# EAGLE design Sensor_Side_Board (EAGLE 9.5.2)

## Sheet 1 of 2: Sensor side expansion board for hoop house controller - Inputs
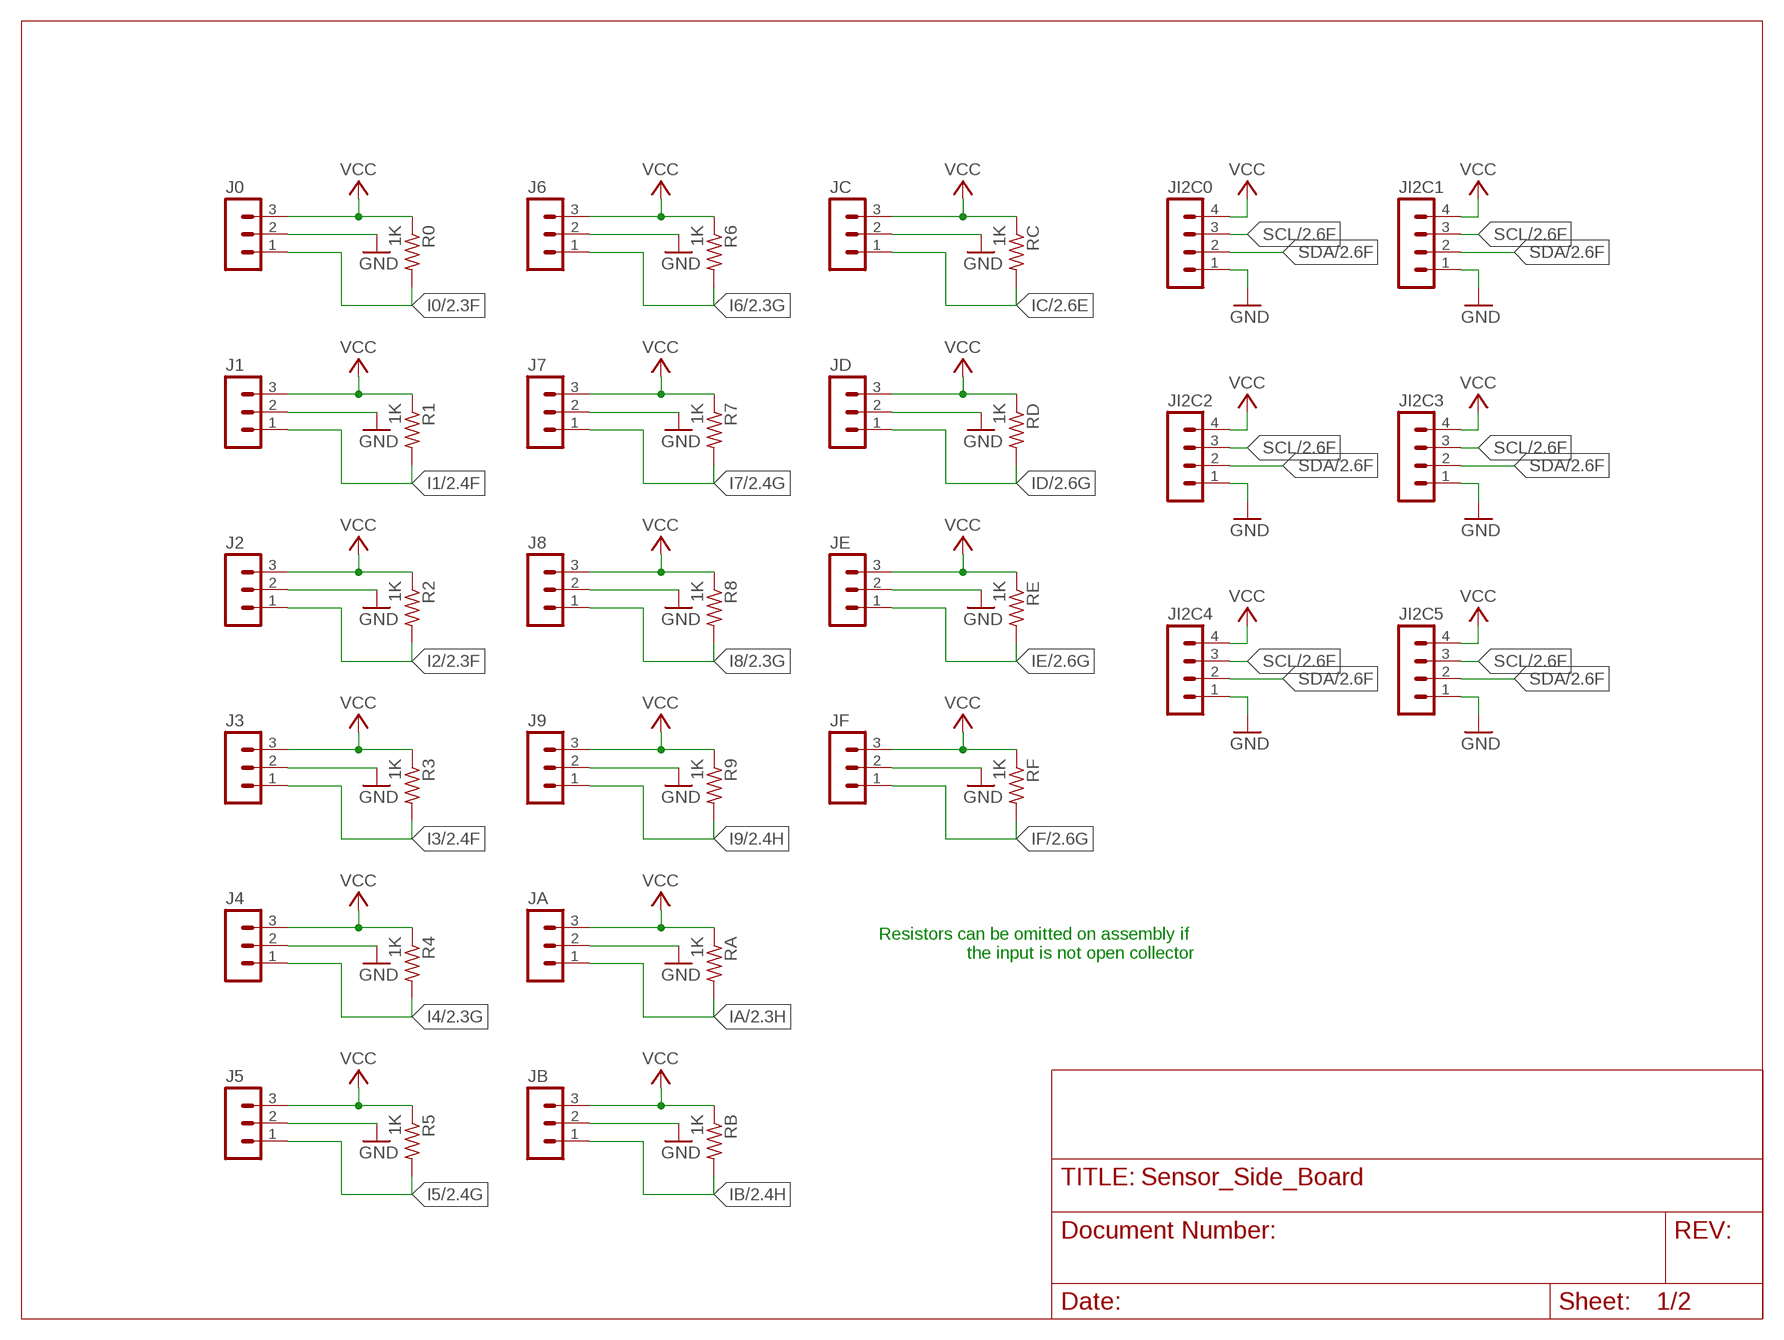
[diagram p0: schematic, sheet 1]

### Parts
J0  MA03-1  [MA03-1]
J1  MA03-1  [MA03-1]
J2  MA03-1  [MA03-1]
J3  MA03-1  [MA03-1]
J4  MA03-1  [MA03-1]
J5  MA03-1  [MA03-1]
J6  MA03-1  [MA03-1]
J7  MA03-1  [MA03-1]
J8  MA03-1  [MA03-1]
J9  MA03-1  [MA03-1]
JA  MA03-1  [MA03-1]
JB  MA03-1  [MA03-1]
JC  MA03-1  [MA03-1]
JD  MA03-1  [MA03-1]
JE  MA03-1  [MA03-1]
JF  MA03-1  [MA03-1]
JI2C0  MA04-1  [MA04-1]
JI2C1  MA04-1  [MA04-1]
JI2C2  MA04-1  [MA04-1]
JI2C3  MA04-1  [MA04-1]
JI2C4  MA04-1  [MA04-1]
JI2C5  MA04-1  [MA04-1]
R0  1K  R-US_0411/15  [0411/15]
R1  1K  R-US_0411/15  [0411/15]
R2  1K  R-US_0411/15  [0411/15]
R3  1K  R-US_0411/15  [0411/15]
R4  1K  R-US_0411/15  [0411/15]
R5  1K  R-US_0411/15  [0411/15]
R6  1K  R-US_0411/15  [0411/15]
R7  1K  R-US_0411/15  [0411/15]
R8  1K  R-US_0411/15  [0411/15]
R9  1K  R-US_0411/15  [0411/15]
RA  1K  R-US_0411/15  [0411/15]
RB  1K  R-US_0411/15  [0411/15]
RC  1K  R-US_0411/15  [0411/15]
RD  1K  R-US_0411/15  [0411/15]
RE  1K  R-US_0411/15  [0411/15]
RF  1K  R-US_0411/15  [0411/15]

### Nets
GND: J0.2 J1.2 J2.2 J3.2 J4.2 J5.2 J6.2 J7.2 J8.2 J9.2 JA.2 JB.2 JC.2 JD.2 JE.2 JF.2 JI2C0.1 JI2C1.1 JI2C2.1 JI2C3.1 JI2C4.1 JI2C5.1 ; also sheet 2
I0: J0.1 R0.2 ; also sheet 2
I1: J1.1 R1.2 ; also sheet 2
I2: J2.1 R2.2 ; also sheet 2
I3: J3.1 R3.2 ; also sheet 2
I4: J4.1 R4.2 ; also sheet 2
I5: J5.1 R5.2 ; also sheet 2
I6: J6.1 R6.2 ; also sheet 2
I7: J7.1 R7.2 ; also sheet 2
I8: J8.1 R8.2 ; also sheet 2
I9: J9.1 R9.2 ; also sheet 2
IA: JA.1 RA.2 ; also sheet 2
IB: JB.1 RB.2 ; also sheet 2
IC: JC.1 RC.2 ; also sheet 2
ID: JD.1 RD.2 ; also sheet 2
IE: JE.1 RE.2 ; also sheet 2
IF: JF.1 RF.2 ; also sheet 2
SCL: JI2C0.3 JI2C1.3 JI2C2.3 JI2C3.3 JI2C4.3 JI2C5.3 ; also sheet 2
SDA: JI2C0.2 JI2C1.2 JI2C2.2 JI2C3.2 JI2C4.2 JI2C5.2 ; also sheet 2
VCC: J0.3 J1.3 J2.3 J3.3 J4.3 J5.3 J6.3 J7.3 J8.3 J9.3 JA.3 JB.3 JC.3 JD.3 JE.3 JF.3 JI2C0.4 JI2C1.4 JI2C2.4 JI2C3.4 JI2C4.4 JI2C5.4 R0.1 R1.1 R2.1 R3.1 R4.1 R5.1 R6.1 R7.1 R8.1 R9.1 RA.1 RB.1 RC.1 RD.1 RE.1 RF.1 ; also sheet 2

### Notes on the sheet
- Resistors can be omitted on assembly if 
  the input is not open collector

## Sheet 2 of 2: Sensor side expansion board for hoop house controller - ESP, optical isolation, and output
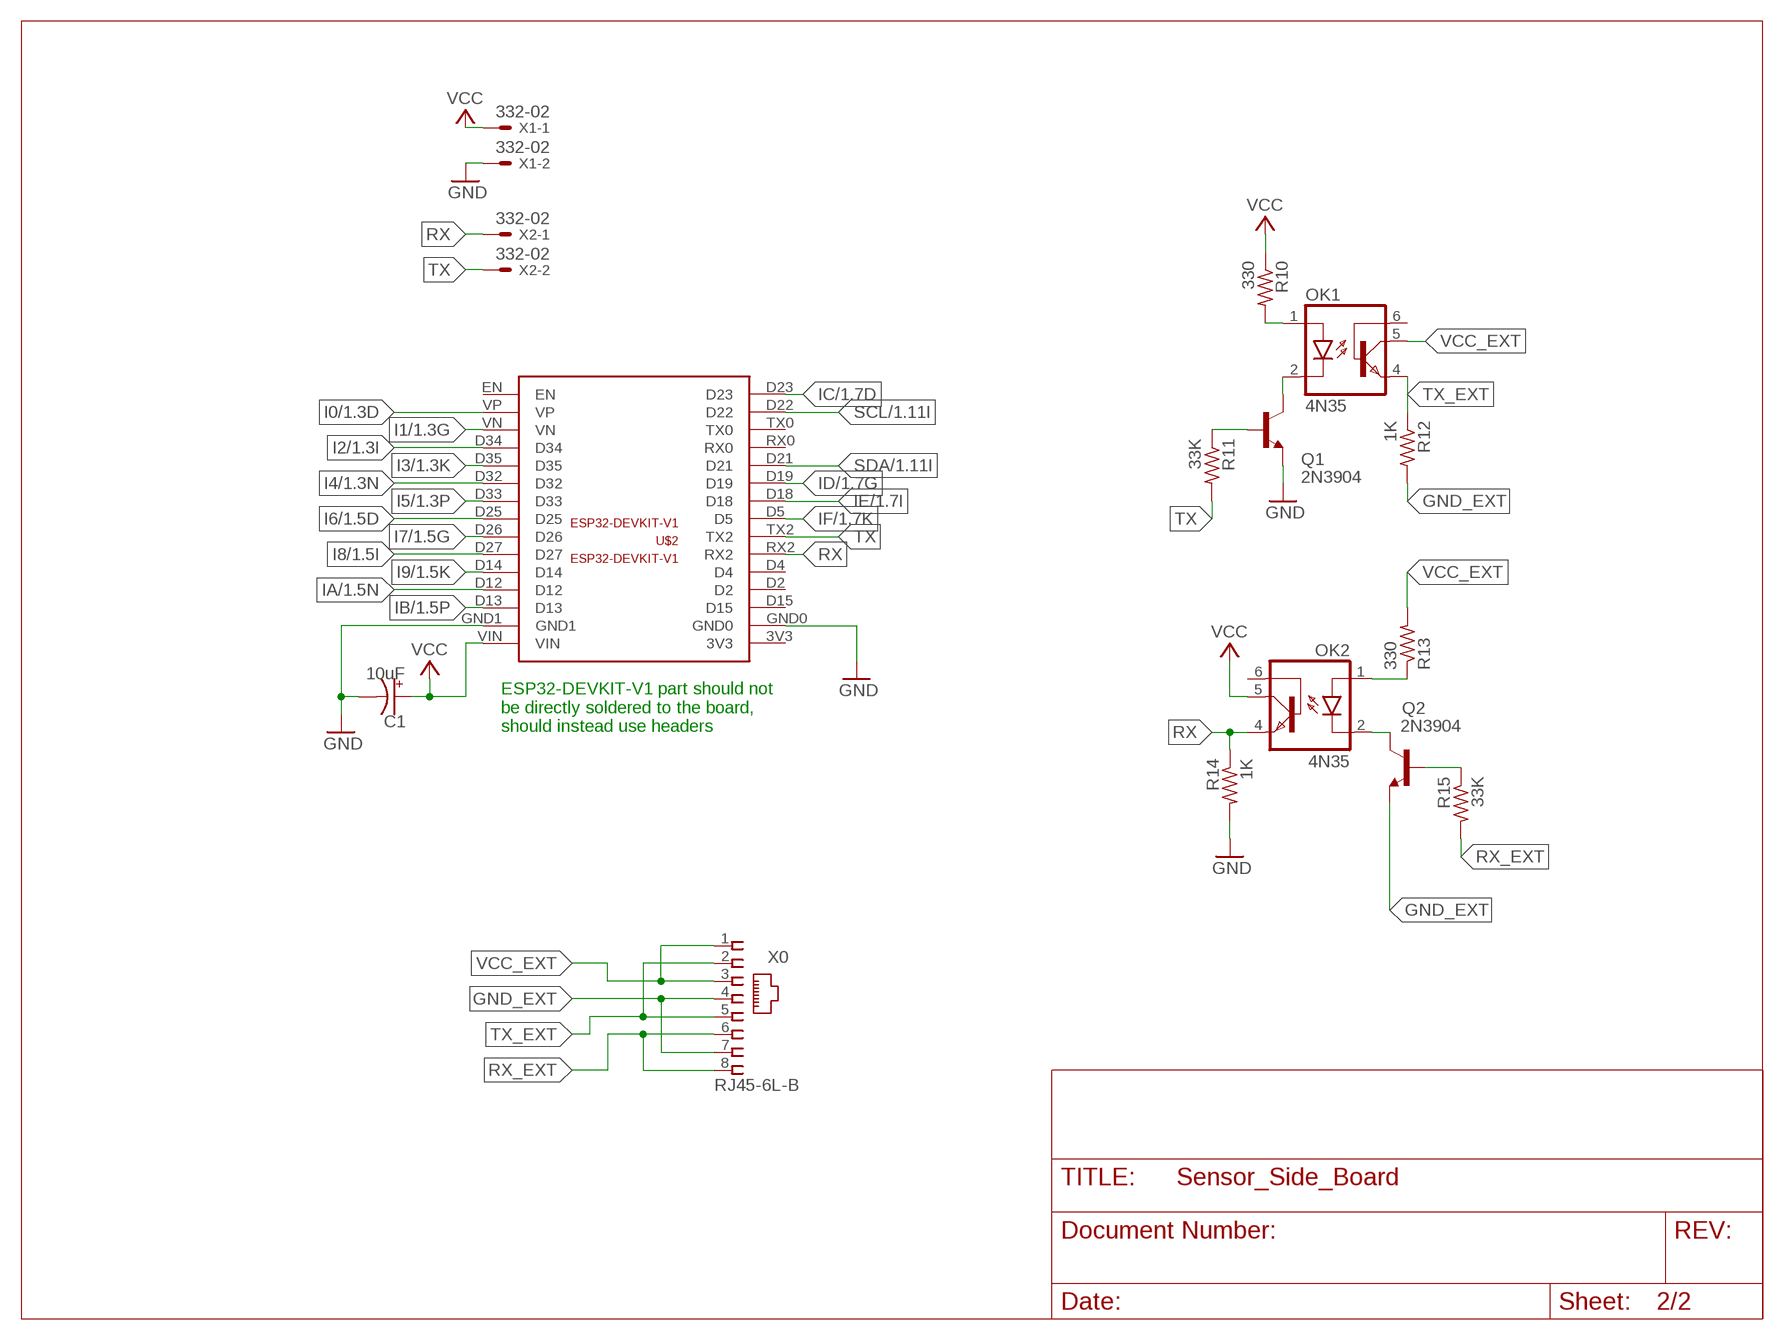
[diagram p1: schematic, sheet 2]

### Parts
C1  10uF  CPOL-USE3.5-10  [E3,5-10]
OK1  4N35  [DIL06]
OK2  4N35  [DIL06]
Q1  2N3904  [TO92]
Q2  2N3904  [TO92]
R10  330  R-US_0411/15  [0411/15]
R11  33K  R-US_0411/15  [0411/15]
R12  1K  R-US_0411/15  [0411/15]
R13  330  R-US_0411/15  [0411/15]
R14  1K  R-US_0411/15  [0411/15]
R15  33K  R-US_0411/15  [0411/15]
U$2  ESP32-DEVKIT-V1  [ESP32-DEVKIT-V1]
X0  RJ45-6L-B  [RJ45-NO-SHIELD]
X1  332-02  [332-02]
X2  332-02  [332-02]

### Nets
GND: C1.- Q1.3(E) R14.2 U$2.GND0 U$2.GND1 X1.2 ; also sheet 1
GND_EXT: Q2.3(E) R12.2 X0.4 X0.7
I0: U$2.VP ; also sheet 1
I1: U$2.VN ; also sheet 1
I2: U$2.D34 ; also sheet 1
I3: U$2.D35 ; also sheet 1
I4: U$2.D32 ; also sheet 1
I5: U$2.D33 ; also sheet 1
I6: U$2.D25 ; also sheet 1
I7: U$2.D26 ; also sheet 1
I8: U$2.D27 ; also sheet 1
I9: U$2.D14 ; also sheet 1
IA: U$2.D12 ; also sheet 1
IB: U$2.D13 ; also sheet 1
IC: U$2.D23 ; also sheet 1
ID: U$2.D19 ; also sheet 1
IE: U$2.D18 ; also sheet 1
IF: U$2.D5 ; also sheet 1
N$6: OK1.1(A) R10.2
N$7: Q1.2(B) R11.1
N$8: OK2.1(A) R13.1
N$9: OK1.2(C) Q1.1(C)
N$13: OK2.2(C) Q2.1(C)
N$14: Q2.2(B) R15.1
RX: OK2.4(EMI) R14.1 U$2.RX2 X2.1
RX_EXT: R15.2 X0.6 X0.8
SCL: U$2.D22 ; also sheet 1
SDA: U$2.D21 ; also sheet 1
TX: R11.2 U$2.TX2 X2.2
TX_EXT: OK1.4(EMI) R12.1 X0.2 X0.5
VCC: C1.+ OK2.5(COL) R10.1 U$2.VIN X1.1 ; also sheet 1
VCC_EXT: OK1.5(COL) R13.2 X0.1 X0.3
Unconnected: OK1.6(BAS) OK2.6(BAS) U$2.3V3 U$2.D2 U$2.D4 U$2.D15 U$2.EN U$2.RX0 U$2.TX0

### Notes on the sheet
- ESP32-DEVKIT-V1 part should not
  be directly soldered to the board,
  should instead use headers

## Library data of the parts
C1 = rcl:CPOL-US: POLARIZED CAPACITOR, American symbol; SPICEPREFIX: C
J0 J1-J9 JA JB JC JD JE JF = con-lstb:MA03-1: PIN HEADER; OC_FARNELL: unknown; OC_NEWARK: unknown
JI2C0 JI2C1-JI2C5 = con-lstb:MA04-1: PIN HEADER; OC_FARNELL: unknown; OC_NEWARK: unknown
OK1 OK2 = optocoupler:4N35: MOTOROLA OPTO COUPLER; MF: FAIRCHILD SEMICONDUCTOR; MPN: 4N35; OC_FARNELL: 1328375; OC_NEWARK: 72K9946
Q1 Q2 = transistor-npn:2N3904: NPN Transistor
R0 R1-R15 RA RB RC RD RE RF = resistor:R-US_: RESISTOR, American symbol
U$2 = FF Hoop House Controller:ESP32-DEVKIT-V1
X0 = con-tycoelectronics:RJ45: CORCOM Modular RJ Jacks No Shield Source: www.tycoelectronics.com .. ENG_DS_1654001_1099_RJ_L_0507.pdf; MPN: RJ45-6L-B; OC_FARNELL: unknown; OC_NEWARK: 16R6090
X1 X2 = con-garry:332-02: 2 Pin - 2mm Dual Row

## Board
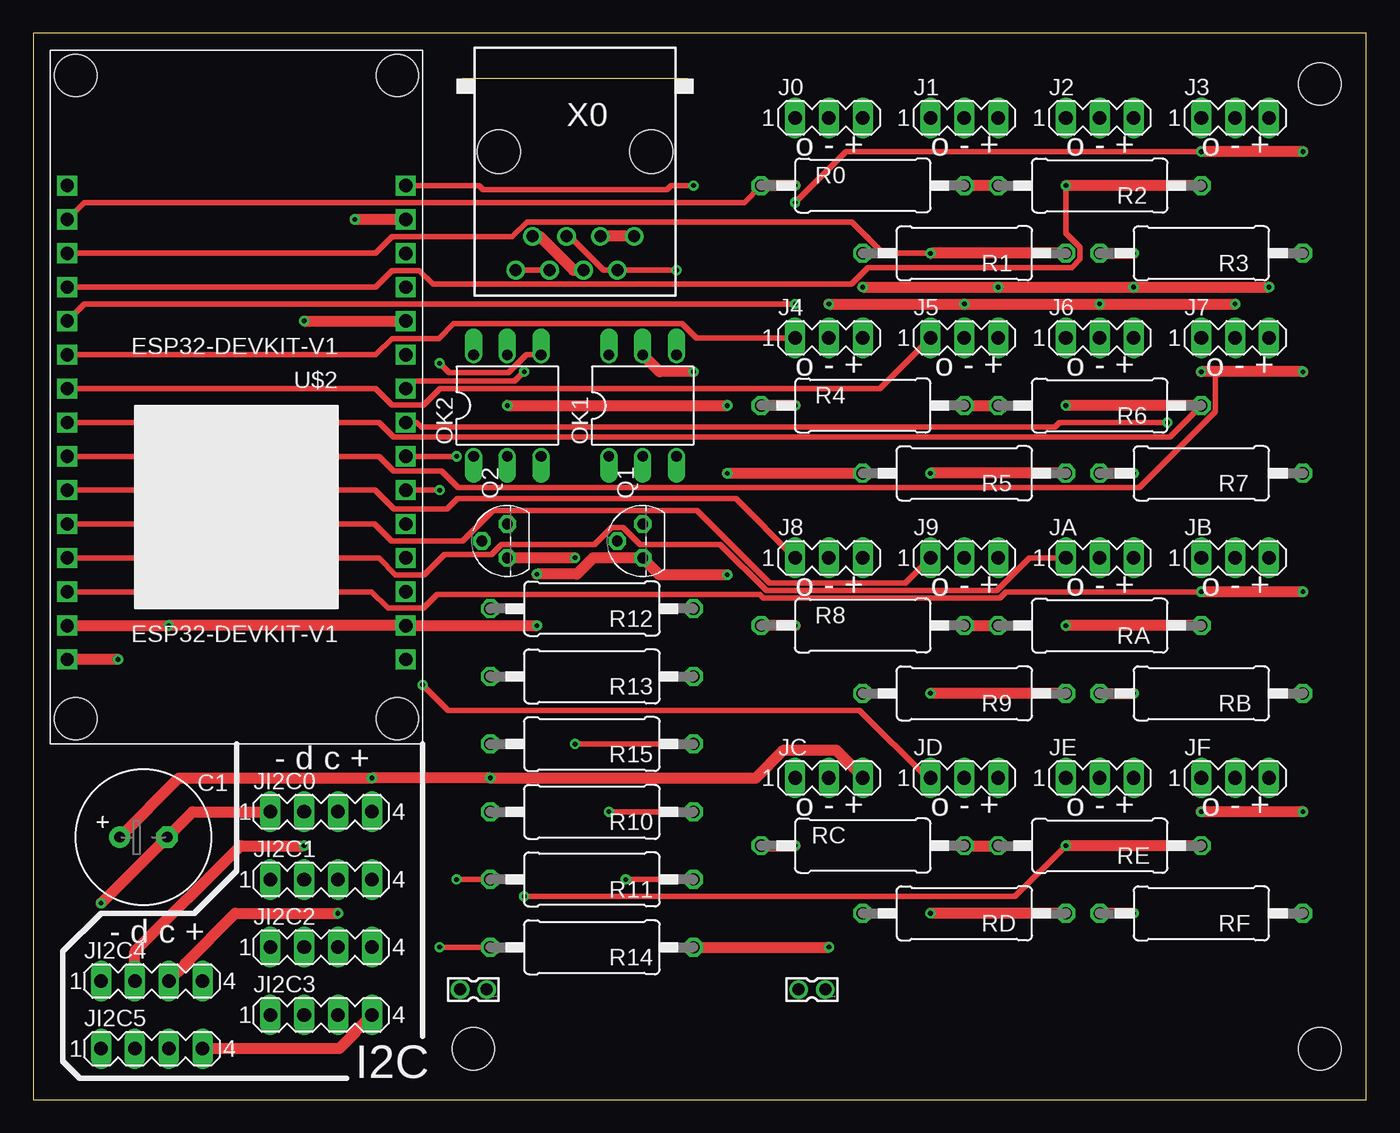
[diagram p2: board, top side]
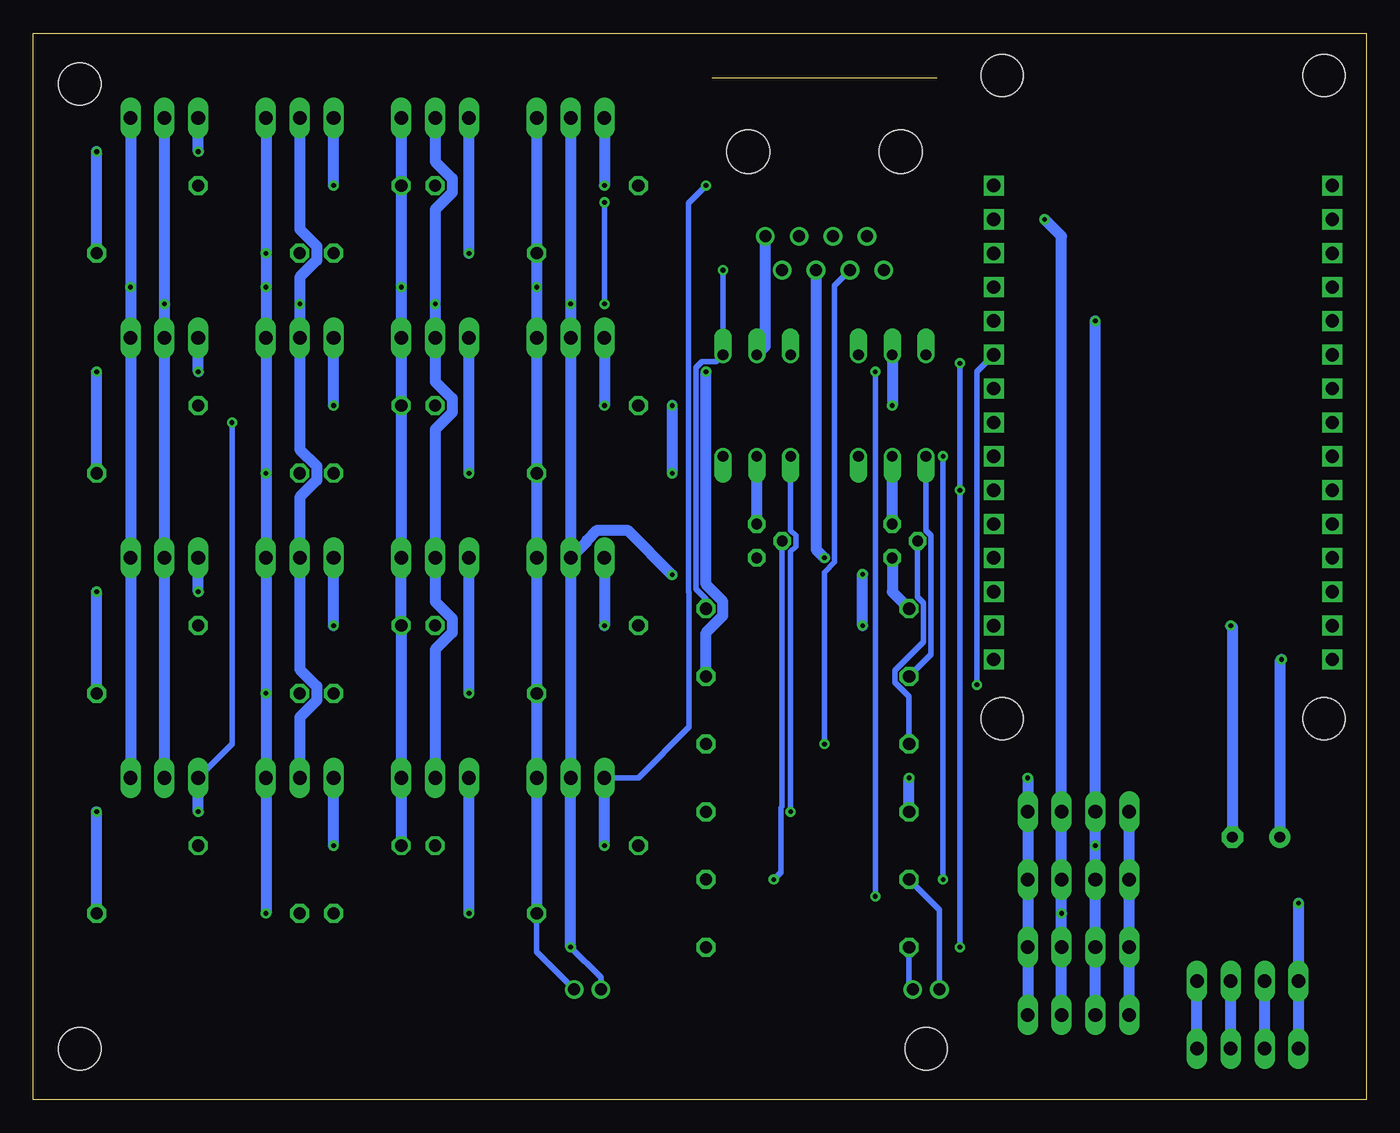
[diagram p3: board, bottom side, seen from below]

Size 100 x 80 mm. Coordinates in mm from the lower left corner, seen from the top.
Outline: 0,0 100,0 100,80 0,80 0,0
Copper layers (1*16): Top 0.035mm / dielectric 1.5mm / Bottom 0.035mm
Design rules "default": minimum track width 6mil, minimum drill 0.35mm, track to track 6mil, track to pad 6mil, pad to pad 6mil, via to via 6mil, smd to smd 6mil, copper to edge 40mil, drill to drill 6mil, minimum pad ring 10mil, minimum via ring 8mil, stop-mask expansion 4mil, vias tented up to drill 0mil, thermal gap 10mil
Holes 3.17 mm at 96.52,3.81 3.17,76.83 96.52,76.2 27.3,76.83 33.02,3.81 3.17,28.57 27.3,28.57

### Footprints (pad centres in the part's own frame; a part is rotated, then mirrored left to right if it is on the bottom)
E3,5-10 = drill 0.813 pad 1.6: + -1.778,0 | drill 0.813 pad 1.6 octagon: - 1.778,0
MA03-1 = drill 1.016 long: 1 -2.54,0; 2 0,0; 3 2.54,0
MA04-1 = drill 1.016 long: 1 -3.81,0; 2 -1.27,0; 3 1.27,0; 4 3.81,0
DIL06 = drill 0.813 offset: 1 -2.54,-3.81; 2 0,-3.81; 3 2.54,-3.81; 4 2.54,3.81; 5 0,3.81; 6 -2.54,3.81
TO92 = drill 0.813 octagon: 1 1.27,0; 2 0,1.905; 3 -1.27,0
0411/15 = drill 0.914 octagon: 1 -7.62,0; 2 7.62,0
ESP32-DEVKIT-V1 = drill 1 square: 3V3 -12.7,17.78; D2 -12.7,10.16; D4 -12.7,7.62; D5 -12.7,0; D12 12.7,10.16; D13 12.7,12.7; D14 12.7,7.62; D15 -12.7,12.7; D18 -12.7,-2.54; D19 -12.7,-5.08; D21 -12.7,-7.62; D22 -12.7,-15.24; D23 -12.7,-17.78; D25 12.7,0; D26 12.7,2.54; D27 12.7,5.08; D32 12.7,-5.08; D33 12.7,-2.54; D34 12.7,-10.16; D35 12.7,-7.62; EN 12.7,-17.78; GND0 -12.7,15.24; GND1 12.7,15.24; RX0 -12.7,-10.16; RX2 -12.7,5.08; TX0 -12.7,-12.7; TX2 -12.7,2.54; VIN 12.7,17.78; VN 12.7,-12.7; VP 12.7,-15.24
RJ45-NO-SHIELD = drill 0.9 pad 1.4: 1 -4.445,6.35; 2 -3.175,8.89; 3 -1.905,6.35; 4 -0.635,8.89; 5 0.635,6.35; 6 1.905,8.89; 7 3.175,6.35; 8 4.445,8.89 | hole 3.251: -5.715,0; 5.715,0
332-02 = drill 0.9 pad 1.27: 1 0,-1; 2 0,1

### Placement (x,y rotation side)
C1  8.26,19.68 0 top
J0  59.69,73.66 0 top
J1  69.85,73.66 0 top
J2  80.01,73.66 0 top
J3  90.17,73.66 0 top
J4  59.69,57.15 0 top
J5  69.85,57.15 0 top
J6  80.01,57.15 0 top
J7  90.17,57.15 0 top
J8  59.69,40.64 0 top
J9  69.85,40.64 0 top
JA  80.01,40.64 0 top
JB  90.17,40.64 0 top
JC  59.69,24.13 0 top
JD  69.85,24.13 0 top
JE  80.01,24.13 0 top
JF  90.17,24.13 0 top
JI2C0  21.59,21.59 0 top
JI2C1  21.59,16.51 0 top
JI2C2  21.59,11.43 0 top
JI2C3  21.59,6.35 0 top
JI2C4  8.89,8.89 0 top
JI2C5  8.89,3.81 0 top
OK1  45.72,52.07 0 top
OK2  35.56,52.07 0 top
Q1  45.72,41.91 90 top
Q2  35.56,41.91 90 top
R0  62.23,68.58 180 top
R1  69.85,63.5 0 top
R2  80.01,68.58 0 top
R3  87.63,63.5 0 top
R4  62.23,52.07 180 top
R5  69.85,46.99 0 top
R6  80.01,52.07 0 top
R7  87.63,46.99 0 top
R8  62.23,35.56 180 top
R9  69.85,30.48 0 top
R10  41.91,21.59 0 top
R11  41.91,16.51 180 top
R12  41.91,36.83 180 top
R13  41.91,31.75 0 top
R14  41.91,11.43 0 top
R15  41.91,26.67 0 top
RA  80.01,35.56 0 top
RB  87.63,30.48 0 top
RC  62.23,19.05 180 top
RD  69.85,13.97 0 top
RE  80.01,19.05 0 top
RF  87.63,13.97 0 top
U$2  15.24,50.8 180 top
X0  40.64,71.12 180 top
X1  58.42,8.26 90 top
X2  33.02,8.26 90 top

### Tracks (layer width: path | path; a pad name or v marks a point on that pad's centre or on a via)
GND  (via drill 0.35)
  Top 0.813: U$2.GND1 v10.16,35.56 U$2.GND0 v37.78,35.56 | JI2C0.1 11.94,21.59 C1.- v5.08,14.73 | R14.2 v59.69,11.43 | v37.78,39.42 40.79,39.42 42.01,40.64 Q1.3 46.99,39.37 v52.07,39.37 | v59.69,59.69 v69.85,59.69 v80.01,59.69 v90.17,59.69
  Bottom 0.406: v59.69,11.43 57.42,9.16 X1.2
  Bottom 0.813: v5.08,14.73 JI2C4.1 JI2C5.1 | v10.16,35.56 10.03,35.43 C1.- | JI2C3.1 JI2C2.1 JI2C1.1 JI2C0.1 | J3.2 v90.17,59.69 J7.2 JB.2 JF.2 | J2.2 80.01,65.3 78.74,64.03 78.74,62.97 80.01,61.7 v80.01,59.69 J6.2 80.01,48.79 78.74,47.52 78.74,46.46 80.01,45.19 JA.2 80.01,32.28 78.74,31.01 78.74,29.95 80.01,28.68 JE.2 | JD.2 69.85,33.76 68.58,35.03 68.58,36.09 69.85,37.36 J9.2 69.85,50.27 68.58,51.54 68.58,52.6 69.85,53.87 J5.2 v69.85,59.69 69.85,66.78 68.58,68.05 68.58,69.11 69.85,70.38 J1.2 | J0.2 v59.69,59.69 J4.2 J8.2 | J8.2 JC.2 v59.69,11.43 | J8.2 58.47,41.86 58.47,41.95 57.7,42.72 55.42,42.72 v52.07,39.37 | v37.78,35.56 v37.78,39.42
GND_EXT  (via drill 0.35)
  Top 0.813: v40.64,40.64 Q2.3 | X0.7 37.99,64.76 40.52,62.23 X0.4
  Bottom 0.813: X0.4 41.27,41.27 v40.64,40.64 | Q2.3 35.56,38.1 R12.2
I0  (via drill 0.35)
  Top 0.406: U$2.VP 3.81,67.31 53.34,67.31 R0.2
  Top 0.813: v57.15,68.58 R0.2
  Bottom 0.813: J0.1 v57.15,68.58
I1  (via drill 0.35)
  Top 0.406: U$2.VN 25.69,63.5 26.92,64.73 35.92,64.73 37.03,65.83 61.41,65.83 63.74,63.5 v67.31,63.5
  Top 0.813: R1.2 v67.31,63.5
  Bottom 0.813: v67.31,63.5 J1.1
I2  (via drill 0.35)
  Top 0.406: U$2.D34 25.69,60.96 26.92,62.19 28.96,62.19 29.98,61.17 61.36,61.17 62.63,62.43 77.91,62.43 78.54,63.06 78.54,63.94 77.47,65.01 v77.47,68.58
  Top 0.813: R2.2 v77.47,68.58
  Bottom 0.813: v77.47,68.58 J2.1
I3  (via drill 0.35)
  Top 0.406: U$2.D35 3.81,59.69 v57.15,59.69 | v57.15,67.31 60.96,71.12 v87.63,71.12
  Top 0.813: v95.25,71.12 v87.63,71.12
  Bottom 0.406: v57.15,59.69 v57.15,67.31
  Bottom 0.813: R3.2 v95.25,71.12 | v87.63,71.12 J3.1
I4  (via drill 0.35)
  Top 0.406: U$2.D32 25.69,55.88 26.92,57.11 30.44,57.11 31.55,58.22 48.68,58.22 49.75,57.15 J4.1
  Top 0.813: v57.15,52.07 R4.2
  Bottom 0.813: J4.1 v57.15,52.07
I5  (via drill 0.35)
  Top 0.406: J5.1 63.5,53.34 30.5,53.34 29.28,52.11 26.92,52.11 25.69,53.34 U$2.D33
  Top 0.813: R5.2 v67.31,46.99
  Bottom 0.813: v67.31,46.99 J5.1
I6  (via drill 0.35)
  Top 0.406: R6.2 85.25,49.69 27.04,49.69 25.93,50.8 U$2.D25
  Top 0.813: R6.2 v77.47,52.07
  Bottom 0.813: v77.47,52.07 J6.1
I7  (via drill 0.35)
  Top 0.406: 88.9,54.61 88.7,54.41 88.7,51.63 82.99,45.92 31.86,45.92 30.64,47.15 27.04,47.15 25.93,48.26 U$2.D26
  Top 0.813: v95.25,54.61 88.9,54.61 v87.63,54.61
  Bottom 0.813: R7.2 v95.25,54.61 | v87.63,54.61 J7.1
I8  (via drill 0.35)
  Top 0.406: J8.1 52.7,45.09 31.84,45.09 31.04,44.29 27.06,44.29 25.63,45.72 U$2.D27
  Top 0.813: v57.15,35.56 R8.2
  Bottom 0.813: J8.1 v57.15,35.56
I9  (via drill 0.35)
  Top 0.406: U$2.D14 25.61,43.18 26.88,41.91 32.22,41.91 34.5,44.2 49.78,44.2 55.22,38.76 65.43,38.76 J9.1
  Top 0.813: R9.2 v67.31,30.48
  Bottom 0.813: v67.31,30.48 J9.1
IA  (via drill 0.35)
  Top 0.406: U$2.D12 25.93,40.64 27.2,39.37 29.32,39.37 30.84,40.89 34.38,40.89 35.14,41.66 42.12,41.66 43.39,42.93 44.24,42.93 45.51,41.66 51.53,41.66 54.99,38.2 72.29,38.2 74.73,40.64 JA.1
  Top 0.813: RA.2 v77.47,35.56
  Bottom 0.813: v77.47,35.56 JA.1
IB  (via drill 0.35)
  Top 0.406: v87.63,38.1 72.98,38.1 72.53,37.64 54.76,37.64 54.5,37.9 30.3,37.9 29.28,36.87 26.6,36.87 25.38,38.1 U$2.D13
  Top 0.813: v95.25,38.1 v87.63,38.1
  Bottom 0.813: RB.2 v95.25,38.1 | v87.63,38.1 JB.1
IC  (via drill 0.35)
  Top 0.406: U$2.D23 33.44,68.58 33.75,68.28 47.53,68.28 47.84,68.58 v49.53,68.58
  Top 0.813: RC.2 v57.15,19.05
  Bottom 0.406: v49.53,68.58 50.85,67.26 50.85,38.08 50.8,38.03 50.8,27.94 54.61,24.13 JC.1
  Bottom 0.813: v57.15,19.05 JC.1
ID  (via drill 0.35)
  Top 0.406: JD.1 67.07,24.13 61.99,29.21 31.11,29.21 v29.21,31.11
  Top 0.813: RD.2 v67.31,13.97
  Bottom 0.406: U$2.D19 29.21,54.61 v29.21,31.11
  Bottom 0.813: v67.31,13.97 JD.1
IE  (via drill 0.35)
  Top 0.406: U$2.D18 27.94,53.47 28.37,53.9 36.12,53.9 v36.83,54.61 | v36.83,15.24 73.66,15.24 v77.47,19.05
  Top 0.813: RE.2 v77.47,19.05
  Bottom 0.406: v36.83,54.61 v36.83,15.24
  Bottom 0.813: v77.47,19.05 JE.1
IF  (via drill 0.35)
  Top 0.406: U$2.D5 28.76,50.8 29.12,50.44 76.64,50.44 76.99,50.8 v85.09,50.8
  Top 0.813: v95.25,21.59 v87.63,21.59
  Bottom 0.406: v85.09,50.8 85.09,26.67 JF.1
  Bottom 0.813: RF.2 v95.25,21.59 | v87.63,21.59 JF.1
N$6  (via drill 0.35)
  Top 0.406: R10.2 v43.18,21.59
  Bottom 0.406: OK1.1 43.18,42.71 42.8,42.33 42.8,41.49 43.18,41.11 v43.18,21.59
N$7  (via drill 0.35)
  Top 0.406: R11.1 v44.45,16.51
  Bottom 0.406: Q1.2 43.81,21.99 43.91,21.89 43.91,17.05 v44.45,16.51
N$8
  Bottom 0.406: OK2.1 33.02,42.71 32.64,42.33 32.64,33.4 R13.1
N$9
  Bottom 0.813: Q1.1 OK1.2
N$13
  Bottom 0.813: Q2.1 OK2.2
N$14
  Bottom 0.406: Q2.2 33.66,37.7 33.22,37.27 33.22,34.33 35.36,32.19 35.36,31.31 34.29,30.24 R15.1
RX  (via drill 0.35)
  Top 0.406: R14.1 v30.48,11.43 | v30.48,45.72 U$2.RX2 | OK2.4 37,55.88 35.66,54.55 31.18,54.55 v30.48,55.24
  Bottom 0.406: v30.48,11.43 v30.48,45.72 v30.48,55.24 | R14.1 34.29,8.53 X2.1
RX_EXT  (via drill 0.35)
  Top 0.406: R15.2 v40.64,26.67 | X0.8 X0.6
  Bottom 0.406: v40.64,26.67 40.64,39.56 39.88,40.32 39.88,61.09 X0.6
SCL  (via drill 0.35)
  Top 0.813: v24.13,66.04 U$2.D22 | JI2C4.3 11.38,10.11 11.38,10.2 15.15,13.97 v22.86,13.97
  Bottom 0.813: JI2C5.3 JI2C4.3 | JI2C3.3 JI2C2.3 v22.86,13.97 JI2C1.3 JI2C0.3 22.86,64.77 v24.13,66.04
SDA  (via drill 0.35)
  Top 0.813: v20.32,58.42 U$2.D21 | JI2C4.2 7.62,11.11 15.56,19.05 v20.32,19.05
  Bottom 0.813: JI2C5.2 JI2C4.2 | JI2C3.2 JI2C2.2 JI2C1.2 v20.32,19.05 JI2C0.2 v20.32,58.42
TX  (via drill 0.35)
  Top 0.406: R11.2 v31.75,16.51 | v31.75,48.26 U$2.TX2
  Bottom 0.406: v31.75,16.51 v31.75,48.26 | R11.2 32.02,14.24 X2.2
TX_EXT  (via drill 0.35)
  Top 0.406: v48.26,62.23 X0.2 42.77,62.23 40.44,64.56 40.22,64.56 X0.5
  Bottom 0.406: v48.26,62.23 OK1.4 48.77,55.37 49.85,55.37 50.29,54.93 50.29,38.31 49.53,37.55 R12.1
VCC  (via drill 0.35)
  Top 0.813: v6.35,33.02 U$2.VIN | C1.+ 10.92,24.13 v25.4,24.13 v34.29,24.13 54.2,24.13 56.28,26.21 60.24,26.21 62.27,24.18 JC.3 | JI2C3.4 24.18,5.13 24.18,5.04 22.95,3.81 JI2C5.4 | R3.1 v82.55,63.5 | R7.1 v82.55,46.99 | RB.1 v82.55,30.48 | RC.1 RE.1 | v82.55,13.97 RF.1 | R2.1 R0.1 | v62.23,60.96 v72.39,60.96 v82.55,60.96 v92.71,60.96 | v35.56,52.07 v52.07,52.07 | v52.07,46.99 R5.1 | R4.1 R6.1 | R8.1 RA.1
  Bottom 0.406: RD.1 62.23,11.06 X1.1
  Bottom 0.813: C1.+ 6.48,32.89 v6.35,33.02 | v25.4,24.13 JI2C0.4 JI2C1.4 JI2C2.4 JI2C3.4 | JI2C5.4 JI2C4.4 | J1.3 R2.1 v72.39,60.96 J5.3 R6.1 J9.3 RA.1 JD.3 RE.1 | J2.3 v82.55,63.5 v82.55,60.96 J6.3 v82.55,46.99 JA.3 v82.55,30.48 JE.3 v82.55,13.97 | J3.3 v92.71,60.96 J7.3 JB.3 JF.3 | RD.1 JC.3 R9.1 J8.3 R5.1 J4.3 v62.23,60.96 R1.1 J0.3 | R10.1 v34.29,24.13 | OK2.5 v35.56,52.07 | v52.07,52.07 v52.07,46.99
VCC_EXT  (via drill 0.35)
  Top 0.813: v49.53,54.61 46.99,54.61 OK1.5 | X0.1 X0.3
  Bottom 0.813: R13.2 49.53,35.03 48.26,36.3 48.26,37.36 49.53,38.63 v49.53,54.61 | OK1.5 45.09,56.52 X0.1

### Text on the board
tNames: o - + | o - + | o - + | o - + | o - + | o - + | o - + | o - + | o - + | o - + | o - + | o - + | - d c + | o - + | o - + | o - + | o - + | - d c + | I2C
tValues: - + | TX RX | 2020 Winter - V0 / University of Washington / EE Capstone / Sensor Board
